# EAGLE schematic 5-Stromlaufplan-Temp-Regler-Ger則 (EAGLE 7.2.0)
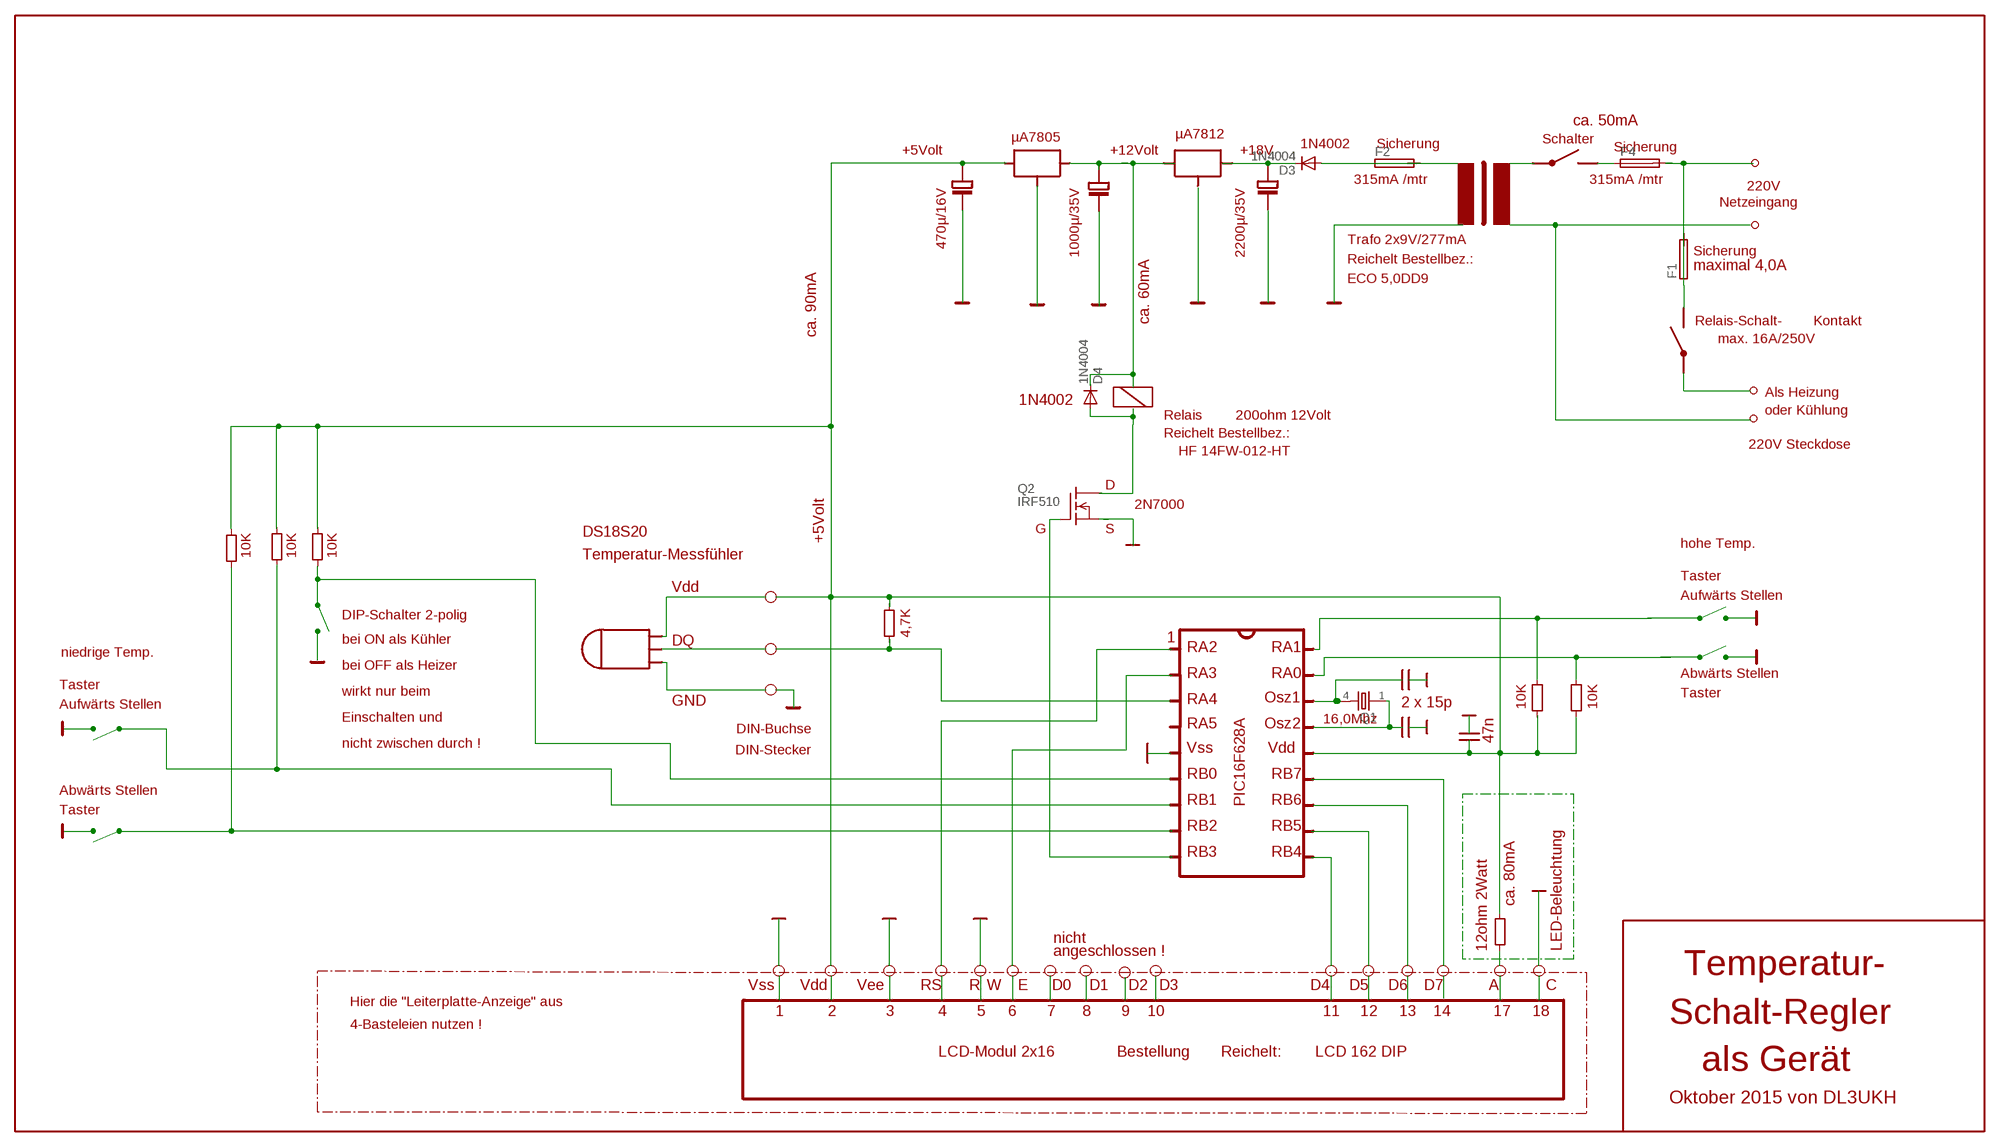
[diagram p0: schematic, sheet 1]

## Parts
D3  1N4004  [DO41-10]
D4  1N4004  [DO41-10]
F1  19559  [19559]
F2  19559  [19559]
F4  19559  [19559]
Q1  86SMX  [86SMX]
Q2  IRF510  [TO220]

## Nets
N$8: Q1.4
N$9: Q1.1
N$31: D4.A
N$48: F1.1 F1.2 F4.2
N$57: D3.C
N$68: Q2.2(D)
N$72: D3.A F2.1 F2.2
N$93: Q2.3(S)
N$94: F4.1
N$96: D4.C
N$97: Q2.1(G)

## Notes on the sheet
- ca. 50mA
- Schalter
- µA7805 | µA7812
- 1N4002 | Sicherung | Sicherung
- +5Volt | +12Volt | +18V
- 315mA /mtr | 315mA /mtr
- 220V
- Netzeingang
- Trafo 2x9V/277mA
- 470µ/16V
- 1000µ/35V | 2200µ/35V | Sicherung
- Reichelt Bestellbez.:
- maximal 4,0A
- ECO 5,0DD9
- ca. 60mA | Relais-Schalt- | Kontakt
- ca. 90mA
- max. 16A/250V
- 1N4002 | Als Heizung
- Relais | 200ohm 12Volt
- oder Kühlung
- Reichelt Bestellbez.:
- HF 14FW-012-HT | 220V Steckdose
- D
- +5Volt
- 2N7000
- DS18S20 | G | S
- hohe Temp.
- 10K | 10K | 10K | Temperatur-Messfühler
- Taster
- Vdd
- Aufwärts Stellen
- DIP-Schalter 2-polig
- 4,7K
- bei ON als Kühler | DQ | 1
- RA2 | RA1
- niedrige Temp.
- bei OFF als Heizer
- RA3 | RA0 | Abwärts Stellen
- Taster
- wirkt nur beim | Taster
- GND | RA4 | Osz1
- Aufwärts Stellen | 2 x 15p | 10K | 10K
- Einschalten und | DIN-Buchse | 16,0Mhz
- RA5 | Osz2
- DIN-Stecker | 47n
- nicht zwischen durch !
- Vss | Vdd
- RB0 | RB7
- Abwärts Stellen
- RB1 | PIC16F628A | RB6
- Taster
- RB2 | RB5
- RB3 | RB4
- ca. 80mA
- nicht
- 12ohm 2Watt | LED-Beleuchtung
- angeschlossen !
- Temperatur-
- Vss | Vdd | Vee | RS | R | W | E | D0 | D1 | D2 | D3 | D4 | D5 | D6 | D7 | A | C
- Hier die "Leiterplatte-Anzeige" aus
- 1 | 2 | 3 | 4 | 5 | 6 | 7 | 8 | 9 | 10 | 11 | 12 | 13 | 14 | 17 | 18
- Schalt-Regler
- 4-Basteleien nutzen !
- LCD-Modul 2x16 | Bestellung | Reichelt: | LCD 162 DIP
- als Gerät
- Oktober 2015 von DL3UKH

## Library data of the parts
D3 D4 = diode:1N4004: DIODE
F1 F2 F4 = fuse:19559: FUSE HOLDER
Q1 = crystal:86SMX: CRYSTAL
Q2 = transistor-fet:IRF510: N-Channel Enhancement MOSFET (HEXFET); 100V; 5,6A; 0,54Ohm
